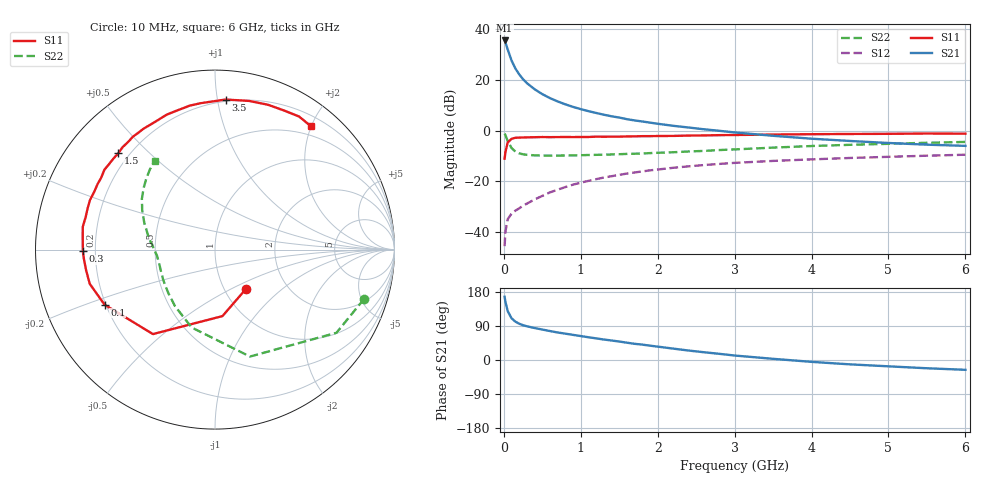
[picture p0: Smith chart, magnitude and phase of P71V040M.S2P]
! SIEMENS Small Signal Semiconductors
! BFP196
! Si NPN RF Bipolar Junction Transistor in SOT143
! VCE = 1 V  IC = 40 mA
! Common Emitter S-Parameters:  May  1996
# GHz  S  MA  R  50
!  f  S11  S21  S12  S22
! GHz  MAG  ANG  MAG  ANG  MAG  ANG  MAG  ANG
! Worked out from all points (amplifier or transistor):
!   36 points, 10 MHz to 6 GHz, reference 50 ohm
!   highest |S21| = 35.7 dB at 10 MHz (marker M1)
!   |S21| within 3 dB of that: start of sweep to 44.17 MHz
!   unconditionally stable (mu >= 1): 436.8 MHz to 5.278 GHz; 5.716 GHz to end of sweep
!   at 250 MHz: K = 0.83, MSG = 25.0 dB, |S12| = -29.7 dB
!   at 1.4 GHz: K = 1.11, MAG = 9.8 dB, |S12| = -18.0 dB
!   at 6 GHz: K = 1.01, MAG = 1.0 dB, |S12| = -9.5 dB
!   S11 on the Smith chart (normalised r, x): 10 MHz: 1.26, -0.60; 100 MHz: 0.20, -0.23; 300 MHz: 0.15, -0.01; 1.5 GHz: 0.16, +0.40; 3.5 GHz: 0.19, +1.06; 6 GHz: 0.35, +1.99
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0.01  0.2787 -51.6  60.66 166.9  0.0052 75.5  0.8751 -18.3
0.02  0.3728 -83.6  55.73 154.0  0.0099 66.1  0.8202 -34.4
0.05  0.5841 -126.3  40.33 129.1  0.0177 50.4  0.6269 -71.9
0.1  0.6876 -153.5  24.38 110.1  0.0229 43.8  0.453 -106.7
0.15  0.7234 -164.7  16.93 101.2  0.0262 44.7  0.3859 -125.3
0.2  0.7275 -171.0  12.94 95.7  0.0291 48.1  0.3556 -136.8
0.25  0.7326 -176.2  10.37 91.8  0.0329 50.1  0.3405 -145.2
0.3  0.7362 -179.3  8.685 89.0  0.0361 52.4  0.333 -150.4
0.4  0.7409 174.2  6.579 84.4  0.0435 55.9  0.3245 -158.1
0.5  0.7474 170.2  5.265 80.4  0.0513 58.2  0.3213 -163.0
0.6  0.7431 165.8  4.394 76.4  0.0602 59.4  0.3204 -166.4
0.7  0.7463 161.8  3.777 72.6  0.0681 59.8  0.3215 -169.1
0.8  0.7493 158.4  3.309 69.5  0.0767 59.7  0.3231 -171.3
1.1  0.75 147.8  2.429 60.0  0.1017 57.9  0.3301 -176.3
1.5  0.7605 135.1  1.814 48.7  0.1337 53.1  0.342 178.7
1.7  0.7709 128.8  1.592 42.7  0.149 50.3  0.3497 175.8
2.2  0.7863 115.1  1.247 30.1  0.1842 43.0  0.3739 169.7
3  0.8196 95.6  0.922 11.8  0.2305 30.9  0.4256 158.3
3.5  0.8382 85.9  0.791 3.1  0.2521 24.1  0.4616 151.5
4.5  0.8594 69.8  0.625 -11.5  0.2883 12.1  0.5246 139.3
5.5  0.8771 57.7  0.528 -21.8  0.3196 1.3  0.5754 129.1
6  0.8707 52.3  0.5 -25.9  0.3342 -4.4  0.5986 124.1
